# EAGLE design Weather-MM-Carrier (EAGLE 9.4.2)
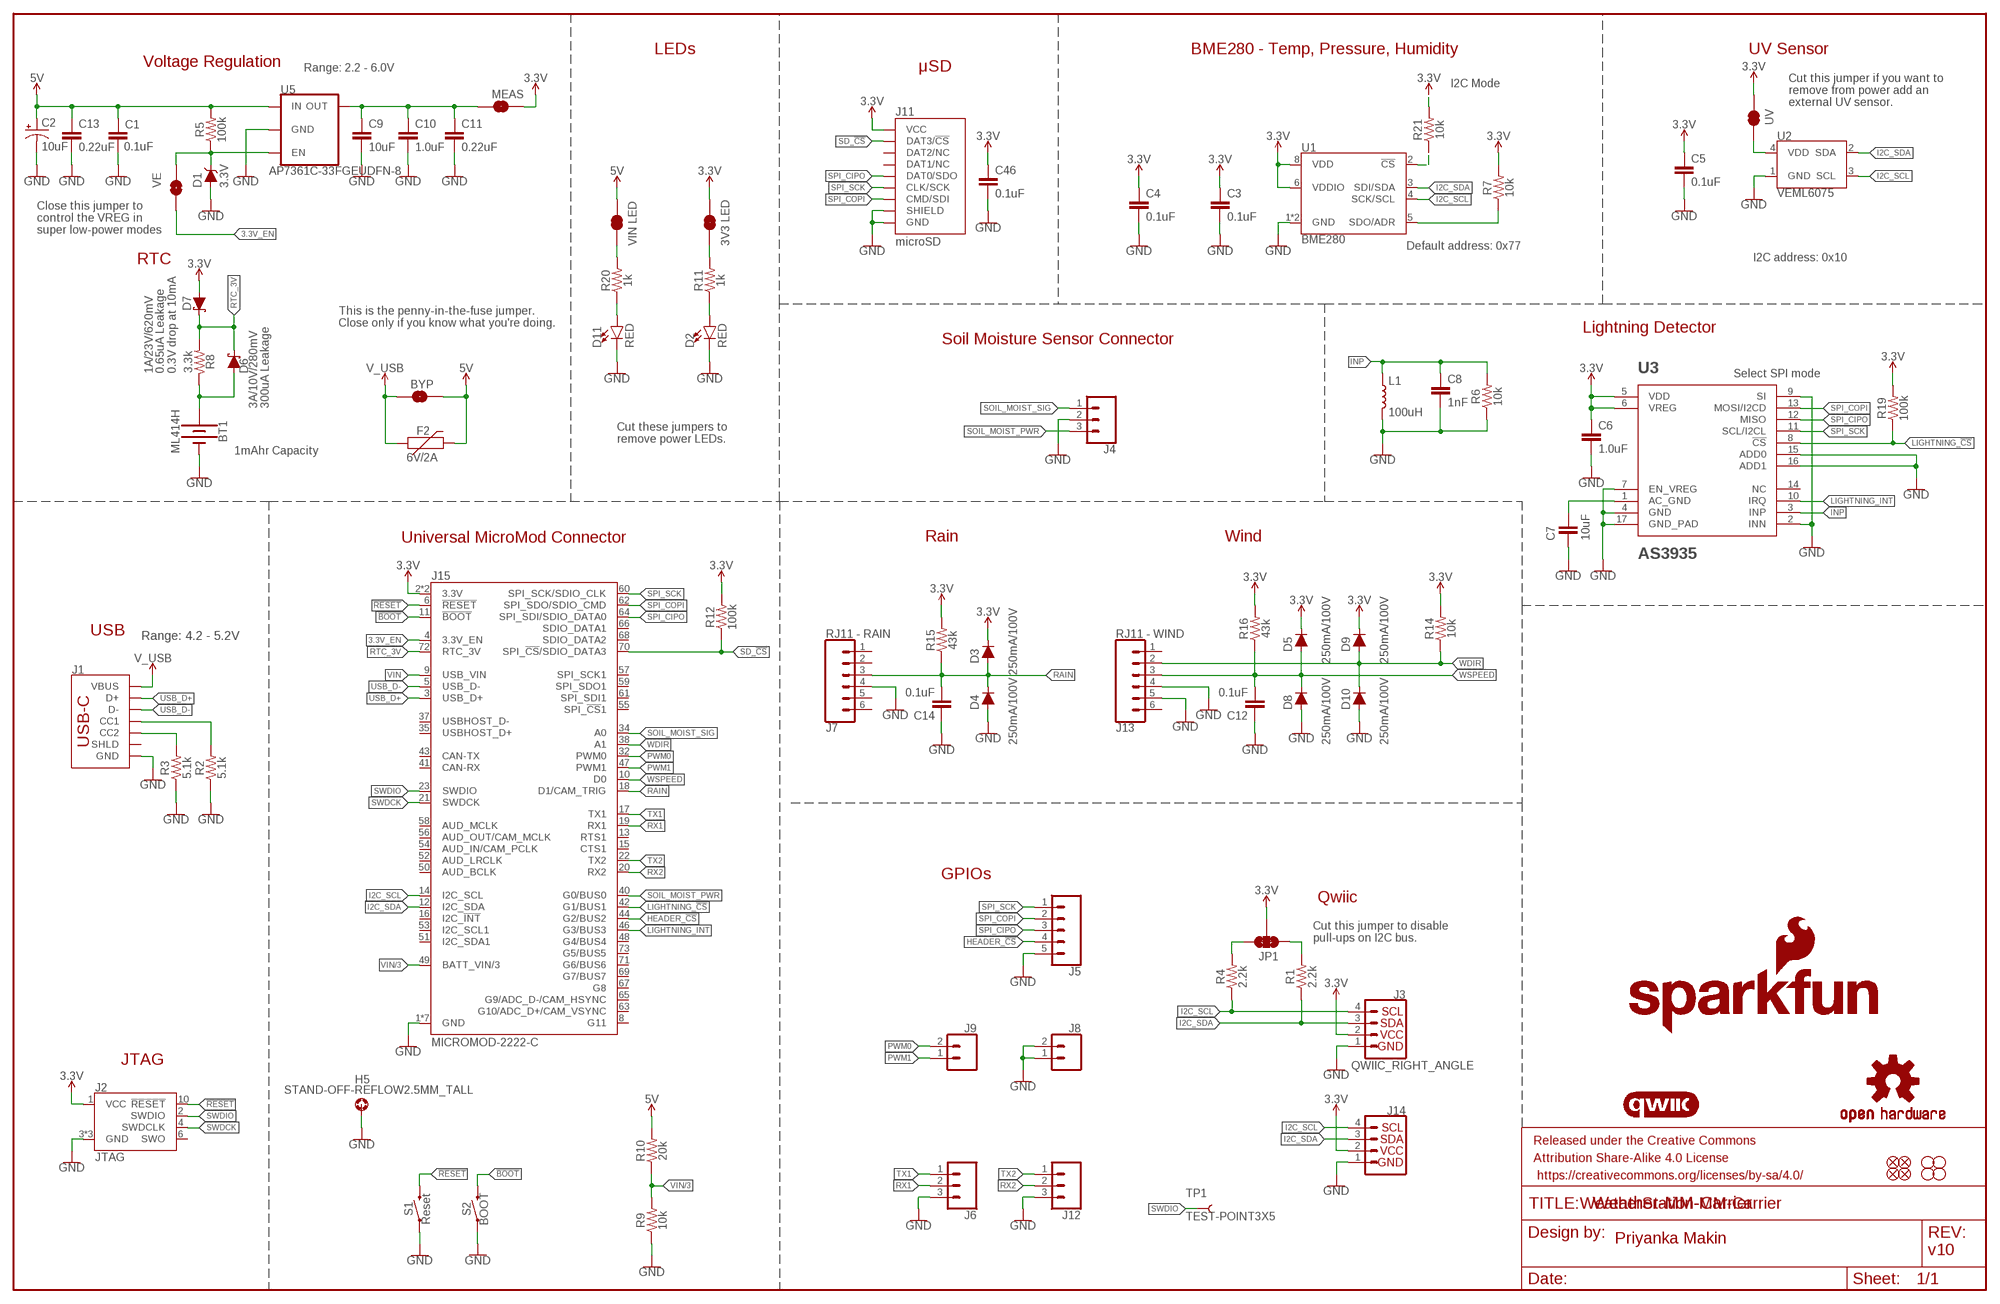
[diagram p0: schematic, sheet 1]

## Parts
BT1  ML414H  ML414H_IV01E_BATTERY  [ML414H_IV01E]
BYP  JUMPER-SMT_2_NO_SILK  [SMT-JUMPER_2_NO_SILK]
C1  0.1uF  0.1UF-0603-25V-(+80/-20%)  [0603]
C2  10uF  10UF-POLAR-EIA3216-16V-10%(TANT)  [EIA3216]
C3  0.1uF  0.1UF-0603-100V-10%  [0603]
C4  0.1uF  0.1UF-0603-100V-10%  [0603]
C5  0.1uF  0.1UF-0603-25V-(+80/-20%)  [0603]
C6  1.0uF  1.0UF-0603-16V-10%  [0603]
C7  10uF  10UF-0603-6.3V-20%  [0603]
C8  1nF  1.0NF/1000PF-0603-50V-10%  [0603]
C9  10uF  10UF-0603-6.3V-20%  [0603]
C10  1.0uF  1.0UF-0603-16V-10%  [0603]
C11  0.22uF  0.22UF-0603-25V-10%  [0603]
C12  0.1uF  0.1UF-0603-25V-(+80/-20%)  [0603]
C13  0.22uF  0.22UF-0603-25V-10%  [0603]
C14  0.1uF  0.1UF-0603-25V-(+80/-20%)  [0603]
C46  0.1uF  0.1UF-0603-25V-(+80/-20%)  [0603]
D1  3.3V  DIODE-ZENER-MM3Z3V3T1G  [SOD-323]
D2  RED  LED-RED0603  [LED-0603]
D3  250mA/100V  DIODE-BAS16J  [SOD-323]
D4  250mA/100V  DIODE-BAS16J  [SOD-323]
D5  250mA/100V  DIODE-BAS16J  [SOD-323]
D6  3A/10V/280mV  DIODE-SCHOTTKY-BAT60A  [SOD-323]
D7  1A/23V/620mV  DIODE-SCHOTTKY-BAT20J  [SOD-323]
D8  250mA/100V  DIODE-BAS16J  [SOD-323]
D9  250mA/100V  DIODE-BAS16J  [SOD-323]
D10  250mA/100V  DIODE-BAS16J  [SOD-323]
D11  RED  LED-RED0603  [LED-0603]
F2  6V/2A  PPTC_6V2A  [1210]
FD1  FIDUCIALUFIDUCIAL  [FIDUCIAL-MICRO]
FD2  FIDUCIALUFIDUCIAL  [FIDUCIAL-MICRO]
FD3  FIDUCIALUFIDUCIAL  [FIDUCIAL-MICRO]
FD4  FIDUCIALUFIDUCIAL  [FIDUCIAL-MICRO]
FRAME1  FRAME-LEDGER  [CREATIVE_COMMONS]
H1  STAND-OFF  [STAND-OFF]
H2  STAND-OFF  [STAND-OFF]
H3  STAND-OFF  [STAND-OFF]
H4  STAND-OFF  [STAND-OFF]
H5  STAND-OFF-REFLOW2.5MM_TALL  [STAND-OFF-REFLOW-M2.5]
J1  USB_C_2-LAYER_PADS  [USB-C-16P-2LAYER-PADS]
J2  JTAG  CORTEX_JTAG_DEBUG_MINIMUM_PTH  [2X5-PTH-1.27MM]
J3  QWIIC_RIGHT_ANGLE  QWIIC_CONNECTORJS-1MM  [JST04_1MM_RA]
J4  CONN_03LATCH  [LATCHTERMINAL-5MM-3]
J5  CONN_05NO_SILK  [1X05_NO_SILK]
J6  CONN_031X03_NO_SILK  [1X03_NO_SILK]
J7  RJ11 - RAIN  RJ11-6  [RJ11-6]
J8  CONN_021X02_NO_SILK  [1X02_NO_SILK]
J9  CONN_021X02_NO_SILK  [1X02_NO_SILK]
J11  microSD  MICRO-SD-SDIOPUSH-PUSH  [MICRO-SD-SOCKET]
J12  CONN_031X03_NO_SILK  [1X03_NO_SILK]
J13  RJ11 - WIND  RJ11-6  [RJ11-6]
J14  I2C_STANDARD_NO_SILK  [1X04_NO_SILK]
J15  MICROMOD-2222-C  [M.2-CONNECTOR-E]
JP1  JUMPER-SMT_3_2-NC_TRACE_SILK  [SMT-JUMPER_3_2-NC_TRACE_SILK]
JP2  VIN LED  JUMPER-SMT_2_NC_TRACE_SILK  [SMT-JUMPER_2_NC_TRACE_SILK]
JP3  UV  JUMPER-SMT_2_NC_TRACE_SILK  [SMT-JUMPER_2_NC_TRACE_SILK]
JP4  3V3 LED  JUMPER-SMT_2_NC_TRACE_SILK  [SMT-JUMPER_2_NC_TRACE_SILK]
JP6  VE  JUMPER-SMT_2_NO_SILK  [SMT-JUMPER_2_NO_SILK]
L1  100uH  MA5532-AE  [MA5532-AE]
LOGO1  SFE_LOGO_NAME_FLAME.2_INCH  [SFE_LOGO_NAME_FLAME_.2]
LOGO2  QWIIC_LOGO_CONNECTOR  [QWIIC_5.5MM]
LOGO3  OSHW-LOGOM  [OSHW-LOGO-M]
MEAS  JUMPER-COMBO_2_NC_TRACE  [COMBO-JUMPER_2_NC_TRACE]
R1  2.2k  2.2KOHM-0603-1/10W-1%  [0603]
R2  5.1k  5.1KOHM5.1KOHM-0603-1/10W-1%  [0603]
R3  5.1k  5.1KOHM5.1KOHM-0603-1/10W-1%  [0603]
R4  2.2k  2.2KOHM-0603-1/10W-1%  [0603]
R5  100k  100KOHM-0603-1/10W-1%  [0603]
R6  10k  10KOHM-0603-1/10W-1%  [0603]
R7  10k  10KOHM-0603-1/10W-1%  [0603]
R8  3.3k  3.3KOHM-0603-1/10W-1%  [0603]
R9  10k  10KOHM-0603-1/10W-1%  [0603]
R10  20k  20KOHM-0603-1/10W-1%  [0603]
R11  1k  1KOHM-0603-1/10W-1%  [0603]
R12  100k  100KOHM-0603-1/10W-1%  [0603]
R14  10k  10KOHM-0603-1/10W-1%  [0603]
R15  43k  43KOHM-0603-1/10W-1%  [0603]
R16  43k  43KOHM-0603-1/10W-1%  [0603]
R19  100k  100KOHM-0603-1/10W-1%  [0603]
R20  1k  1KOHM-0603-1/10W-1%  [0603]
R21  10k  10KOHM-0603-1/10W-1%  [0603]
S1  Reset  MOMENTARY-SWITCH-SPST-SMD-5.2-TALL-REDUNDANT  [TACTILE_SWITCH_SMD_5.2MM]
S2  BOOT  MOMENTARY-SWITCH-SPST-SMD-5.2-TALL-REDUNDANT  [TACTILE_SWITCH_SMD_5.2MM]
TP1  TEST-POINT3X5  [PAD.03X.05]
U1  BME280  [LGA-8-2.5X2.5]
U2  VEML6075  [VEML6075_A3OP]
U3  AS3935  AS3935QFN  [16LD_MLPQ]
U5  AP7361C-33FGEUDFN-8  [UDFN-8]

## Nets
3.3V: C3.1 C4.1 C5.1 C6.1 C46.1 D3.C D5.C D7.A D9.C J2.1(VCC) J3.2 J11.VCC J14.2 J15.2(3.3V) J15.74(3.3V) JP1.2 JP3.2 JP4.2 MEAS.2 MEAS.4 R7.2 R12.2 R14.2 R15.2 R16.2 R19.2 R21.2 U1.6(VDDIO) U1.8(VDD) U3.5(VDD) U3.6(VREG)
3.3V_EN: J15.4(3.3V_EN) JP6.1
!BOOT!: J15.11(!BOOT!) S2.3 S2.4
!RESET!: J2.10(!RESET) J15.6(!RESET!) S1.3 S1.4
GND: BT1.- C1.2 C2.- C3.2 C4.2 C5.2 C6.2 C7.2 C8.2 C9.2 C10.2 C11.2 C12.1 C13.2 C14.1 C46.2 D1.A D2.C D4.A D8.A D10.A D11.C H5.1 J1.GND J1.GND2(GND) J2.3(GND) J2.5(GND) J2.9(GND) J3.1 J4.2 J5.5 J6.3 J7.4 J8.1 J8.2 J11.CD1(SHIELD) J11.GND J11.GND1(GND) J11.GND3(GND) J12.3 J13.4 J13.5 J14.1 J15.1(GND) J15.7(GND) J15.33(GND) J15.36(GND) J15.39(GND) J15.45(GND) J15.75(GND) L1.2 R2.1 R3.1 R6.1 R9.1 S1.1 S1.2 S2.1 S2.2 U1.1(GND) U1.7(GND) U2.1(GND) U3.2(INN) U3.4(GND) U3.7(EN_VREG) U3.9(SI) U3.15(ADD0) U3.16(ADD1) U3.17(GND_PAD) U5.4(GND) U5.EP(GND)
HEADER_!CS!: J5.4 J15.44(G2/BUS2)
I2C_SCL: J3.4 J14.4 J15.14(I2C_SCL) R4.1 U1.4(SCK/SCL) U2.3(SCL)
I2C_SDA: J3.3 J14.3 J15.12(I2C_SDA) R1.1 U1.3(SDI/SDA) U2.2(SDA)
INP: C8.1 L1.1 R6.2 U3.3(INP)
LIGHTNING_!CS!: J15.42(G1/BUS1) R19.1 U3.8(!CS)
LIGHTNING_INT: J15.46(G3/BUS3) U3.10(IRQ)
N$1: C9.1 C10.1 C11.1 MEAS.1 MEAS.3 U5.1(OUT)
N$2: JP1.3 R4.2
N$3: JP1.1 R1.2
N$4: JP4.1 R11.2
N$5: JP2.1 R20.2
N$6: D2.A R11.1
N$7: JP3.1 U2.4(VDD)
N$8: R7.1 U1.5(SDO/ADR)
N$10: J1.A5(CC1) R2.2
N$11: J1.B5(CC2) R3.2
N$14: BT1.+ D6.A R8.1
N$15: C7.1 U3.1(AC_GND)
N$16: D11.A R20.1
N$19: R21.1 U1.2(!CS)
PWM0: J9.2 J15.32(PWM0)
PWM1: J9.1 J15.47(PWM1)
RAIN: C14.2 D3.A D4.C J7.3 J15.18(D1/CAM_TRIG) R15.1
RTC_3V: D6.C D7.C J15.72(RTC_3V) R8.2
RX1: J6.2 J15.19(RX1)
RX2: J12.2 J15.20(RX2)
SD_!CS!: J11.CS/DAT3(DAT3/!CS!) J15.70(SPI_!CS!/SDIO_DATA3) R12.1
SOIL_MOIST_PWR: J4.3 J15.40(G0/BUS0)
SOIL_MOIST_SIG: J4.1 J15.34(A0)
SPI_CIPO: J5.3 J11.DO/DAT0(DAT0/SDO) J15.64(SPI_SDI/SDIO_DATA0) U3.12(MISO)
SPI_COPI: J5.2 J11.DI/CMD(CMD/SDI) J15.62(SPI_SDO/SDIO_CMD) U3.13(MOSI/I2CD)
SPI_SCK: J5.1 J11.SCLK(CLK/SCK) J15.60(SPI_SCK/SDIO_CLK) U3.11(SCL/I2CL)
SWDCK: J2.4(SWDCLK) J15.21(SWDCK)
SWDIO: J2.2(SWDIO) J15.23(SWDIO) TP1.P$1
TX1: J6.1 J15.17(TX1)
TX2: J12.1 J15.22(TX2)
USB_D+: J1.A6(D+) J1.B6(D+) J15.3(USB_D+)
USB_D-: J1.A7(D-) J1.B7(D-) J15.5(USB_D-)
V_USB: BYP.1 F2.1 J1.VBUS1(VBUS) J1.VBUS2(VBUS)
VIN: BYP.2 C1.1 C2.+ C13.1 F2.2 J15.9(USB_VIN) JP2.2 R5.2 R10.2 U5.8(IN) ; supply symbol labelled 5V
VIN/3: J15.49(BATT_VIN/3) R9.2 R10.1
VREG_EN: D1.C JP6.2 R5.1 U5.5(EN)
WDIR: D9.A D10.C J13.2 J15.38(A1) R14.1
WSPEED: C12.2 D5.A D8.C J13.3 J15.10(D0) R16.1
Unconnected: J1.SHLD1(SHLD) J1.SHLD2(SHLD) J1.SHLD3(SHLD) J1.SHLD4(SHLD) J2.6(SWO) J7.1 J7.2 J7.5 J7.6 J11.DAT1(DAT1/NC) J11.DAT2(DAT2/NC) J13.1 J13.6 J15.8(G11) J15.13(RTS1) J15.15(CTS1) J15.16(I2C_!INT!) J15.35(USBHOST_D+) J15.37(USBHOST_D-) J15.41(CAN-RX) J15.43(CAN-TX) J15.48(G4/BUS4) J15.50(AUD_BCLK) J15.51(I2C_SDA1) J15.52(AUD_LRCLK) J15.53(I2C_SCL1) J15.54(AUD_IN/CAM_PCLK) J15.55(SPI_!CS!1) J15.56(AUD_OUT/CAM_MCLK) J15.57(SPI_SCK1) J15.58(AUD_MCLK) J15.59(SPI_SDO1) J15.61(SPI_SDI1) J15.63(G10/ADC_D+/CAM_VSYNC) J15.65(G9/ADC_D-/CAM_HSYNC) J15.66(SDIO_DATA1) J15.67(G8) J15.68(SDIO_DATA2) J15.69(G7/BUS7) J15.71(G6/BUS6) J15.73(G5/BUS5) U3.14(NC)

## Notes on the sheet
- LEDs | BME280 - Temp, Pressure, Humidity | UV Sensor
- Voltage Regulation
- Range: 2.2 - 6.0V | μSD
- I2C Mode
- Cut this jumper if you want to
  remove from power add an 
  external UV sensor.
- Close this jumper to 
  control the VREG in 
  super low-power modes
- Default address: 0x77
- RTC | I2C address: 0x10
- This is the penny-in-the-fuse jumper.
  Close only if you know what you're doing.
- Lightning Detector
- Soil Moisture Sensor Connector
- 0.65uA Leakage
  0.3V drop at 10mA
- Select SPI mode
- 300uA Leakage
- Cut these jumpers to
  remove power LEDs.
- 1mAhr Capacity
- Universal MicroMod Connector | Rain | Wind
- USB
- Range: 4.2 - 5.2V
- GPIOs
- Qwiic
- Cut this jumper to disable
  pull-ups on I2C bus.
- JTAG
- WeatherStation-MM-Carrier
- Priyanka Makin
- v10

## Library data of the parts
BT1 = SparkFun-Batteries:ML414H_IV01E_BATTERY: SEIKO ML414H-IV01E Reflowable Lithium Battery; PROD_ID: BATT-14267
BYP JP6 = SparkFun-Jumpers:JUMPER-SMT_2_NO: Normally open jumper
C1 C5 C12 C14 C46 = SparkFun-Capacitors:0.1UF: 0.1µF ceramic capacitors; PROD_ID: CAP-00810
C2 = SparkFun-Capacitors:10UF-POLAR: 10.0µF polarized capacitors; PROD_ID: CAP-00811
C3 C4 = SparkFun-Capacitors:0.1UF: 0.1µF ceramic capacitors; PROD_ID: CAP-08390
C6 C10 = SparkFun-Capacitors:1.0UF: 1µF ceramic capacitors; PROD_ID: CAP-00868
C7 C9 = SparkFun-Capacitors:10UF: 10.0µF ceramic capacitors; PROD_ID: CAP-11015
C8 = SparkFun-Capacitors:1.0NF/1000PF: 1nF/1,000pF ceramic capacitors; PROD_ID: CAP-07886
C11 C13 = SparkFun-Capacitors:0.22UF: 0.22µF ceramic capacitors; PROD_ID: CAP-07822
D1 = SparkFun-DiscreteSemi:DIODE-ZENER: Zener Diode; PROD_ID: DIO-11284
D2 D11 = SparkFun-LED:LED-RED: Red SMD LED; PROD_ID: DIO-00819
D3-D5 D8-D10 = SparkFun-DiscreteSemi:DIODE: Diode; PROD_ID: DIO-09646
D6 = SparkFun-DiscreteSemi:DIODE-SCHOTTKY: Schottky diode; PROD_ID: DIO-14072
D7 = SparkFun-DiscreteSemi:DIODE-SCHOTTKY: Schottky diode; PROD_ID: DIO-11623
F2 = SparkFun-Fuses:PPTC: Resettable Fuse PPTC; PROD_ID: RES-14313
FD1-FD4 = SparkFun-Aesthetics:FIDUCIAL: Fiducial Alignment Points
FRAME1 = SparkFun-Aesthetics:FRAME-LEDGER: Schematic Frame - Ledger
H1-H4 = SparkFun-Hardware:STAND-OFF: Stand Off
H5 = SparkFun-Hardware:STAND-OFF-REFLOW: Stand Off Reflow Compatible; PROD_ID: HW-14899
J1 = SparkFun-Connectors:USB_C: USB Type C 16Pin Connector Super Speed pins not available on the 16-pin purely SMD connector so this part is best for USB 2.0 implementations. D1 and D2 are tied together enabling D+/- no matter which way the cable is plugged into the connector. The two channel configuration pins (CC1/2) are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; PROD_ID: CONN-14122
J2 = SparkFun-Connectors:CORTEX_JTAG_DEBUG_MINIMUM: Cortex Debug Connector - 10 pin Supports JTAG debug, Serial Wire debug, and Serial Wire Viewer. PTH and SMD connector options available. General Connector Information Products: PTH Connector -via Digi-Key SparkFun PSoc SparkFun T
J3 = SparkFun-Connectors:QWIIC_CONNECTOR: SparkFun I2C Standard Qwiic Connector An SMD 1mm pitch JST connector makes it easy and quick (get it? Qwiic?) to connect I2C devices to each other. The Qwiic system enables fast and solderless connection between popular platforms and various sensors and actuators. We carry 200mm, 100mm, 50mm, and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; PROD_ID: CONN-13694
J4 = SparkFun-Connectors:CONN_03: Multi connection point. Often used as Generic Header-pin footprint for 0.1 inch spaced/style header connections On any of the 0.1 inch spaced packages, you can populate with these: Break Away Headers - Straight (PRT-00116) Break Away Male Headers - Right Angle (PRT-00553) Female Headers (PRT-00115)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; PROD_ID: CONN-14721
J5 = SparkFun-Connectors:CONN_05: Multi connection point. Often used as Generic Header-pin footprint for 0.1 inch spaced/style header connections On any of the 0.1 inch spaced packages, you can populate with these: Break Away Headers - Straight (PRT-00116) Break Away Male Headers - Right Angle (PRT-00553) Female Headers (PRT-00115)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
J6 J12 = SparkFun-Connectors:CONN_03: Multi connection point. Often used as Generic Header-pin footprint for 0.1 inch spaced/style header connections On any of the 0.1 inch spaced packages, you can populate with these: Break Away Headers - Straight (PRT-00116) Break Away Male Headers - Right Angle (PRT-00553) Female Headers (PRT-00115)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
J7 J13 = SparkFun-Connectors:RJ11-6: RJ11 Jack - 6 pin Commonly found on CAT3 devices and some Microchip programmers. Here is the connector we sell at SparkFun: RJ11 6-Pin Connector (PRT-00132) Datasheet It is used on this SparkFun product: SparkFun Weather Shield (DEV-12081) Weather Meters (SEN-08942); PROD_ID: CONN-08590; SF_ID: PRT-00132; VALUE: RJ11
J8 J9 = SparkFun-Connectors:CONN_02: Multi connection point. Often used as Generic Header-pin footprint for 0.1 inch spaced/style header connections
J11 = SparkFun-Connectors:MICRO-SD-SDIO: microSD Socket for Transflash Push-push type µSD socket. tDoc lines correctly indicate media card edge positions when inserting (unlocked, locked, depressed). NOTE: CD1 and CD2 are connected internally, and the default detect state of the socket is detect pin to ground. SparkFun Products: WAV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; PROD_ID: CONN-07820
J14 = SparkFun-Connectors:I2C_STANDARD: SparkFun I2C Standard Pinout Header SparkFun has standardized on a pinout for all I2C based sensor breakouts. This pinout allows I2C boards to be plugged directly into the headers on Arduino Uno compatible boards, and to be daisy chained easily. Example SparkFun Products: SparkFun Atmospheric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
J15 = SparkFun-MicroMod:MICROMOD: MicroMod Connector Description: A card edge connector and mating PCB connector to allow various MicroMod Processor Boards to be coupled with various carrier boards of different capabilities. Based on the M.2 standard.; PROD_ID: CONN-14877
JP1 = SparkFun-Jumpers:JUMPER-SMT_3_2-NC_TRACE: Normally closed trace jumper (2 of 2 connections) This jumper has a trace between all three pads so they are normally closed (NC). Use a razor knife to open the connection(s). For best results follow the IPC guidelines for cutting traces: Cutout at least 0.063 mm (0.005 in). Remove all loose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
JP2-JP4 = SparkFun-Jumpers:JUMPER-SMT_2_NC_TRACE: Normally closed trace jumper
L1 = SparkFun-Coils:MA5532-AE: RFID Transponder Coil - MA5532-AE; PROD_ID: NDUC-11334
LOGO1 = SparkFun-Aesthetics:SFE_LOGO_NAME_FLAME: SparkFun Font Logo w/ Flame
LOGO2 = SparkFun-Aesthetics:QWIIC_LOGO: Qwiic Logos for placement on schematic and PCB. The 5.5mm silk logo is best for placing next to Qwiic connector.
LOGO3 = SparkFun-Aesthetics:OSHW-LOGO: Open-Source Hardware (OSHW) Logo
MEAS = SparkFun-Jumpers:JUMPER-COMBO_2_NC_TRACE
R1 R4 = SparkFun-Resistors:2.2KOHM: 2.2kΩ resistor; PROD_ID: RES-08272
R2 R3 = SparkFun-Resistors:5.1KOHM; PROD_ID: RES-12083
R5 R12 R19 = SparkFun-Resistors:100KOHM: 100kΩ resistor; PROD_ID: RES-07828
R6 R7 R9 R14 R21 = SparkFun-Resistors:10KOHM: 10kΩ resistor; PROD_ID: RES-00824
R8 = SparkFun-Resistors:3.3KOHM: 3.3kΩ resistor; PROD_ID: RES-07851
R10 = SparkFun-Resistors:20KOHM: 20kΩ resistor; PROD_ID: RES-09383
R11 R20 = SparkFun-Resistors:1KOHM: 1kΩ resistor; PROD_ID: RES-07856
R15 R16 = SparkFun-Resistors:43KOHM: 43kΩ resistor; PROD_ID: RES-07858
S1 S2 = SparkFun-Switches:MOMENTARY-SWITCH-SPST: Momentary Switch (Pushbutton) - SPST; PROD_ID: SWCH-14139
TP1 = SparkFun-Connectors:TEST-POINT: SparkFun Test Points
U1 = SparkFun-Sensors:BME280: Bosch BME280 &ndash; Combined Humidity and Pressure Sensor The BME280 is as combined digital humidity, pressure and temperature sensor based on proven sensing principles. The sensor module is housed in an extremely compact metal-lid LGA package with a footprint of only 2.5×2.5mm² with a height of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; PROD_ID: IC-13090
U2 = SparkFun-Sensors:VEML6075: Vishay VEML6075 UVA and UVB light sensor with I2C interface.; PROD_ID: IC-14149
U3 = SparkFun-Sensors:AS3935: AS3935 Franklin Lightning Sensor The AS3935 is a programmable fully integrated Lightning Sensor IC that detects the presence and approach of potentially hazardous lightning activity in the vicinity and provides an estimation on the distance to the head of the storm. The embedded lightning algorithm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; PROD_ID: IC-11333
U5 = SparkFun-IC-Power:AP7361C-33FGE: AP7361C 3.3V LDO Regulator; PROD_ID: VREG-14094

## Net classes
0 default: width 0 mm, drill 0 mm
1 power: width 0.762 mm

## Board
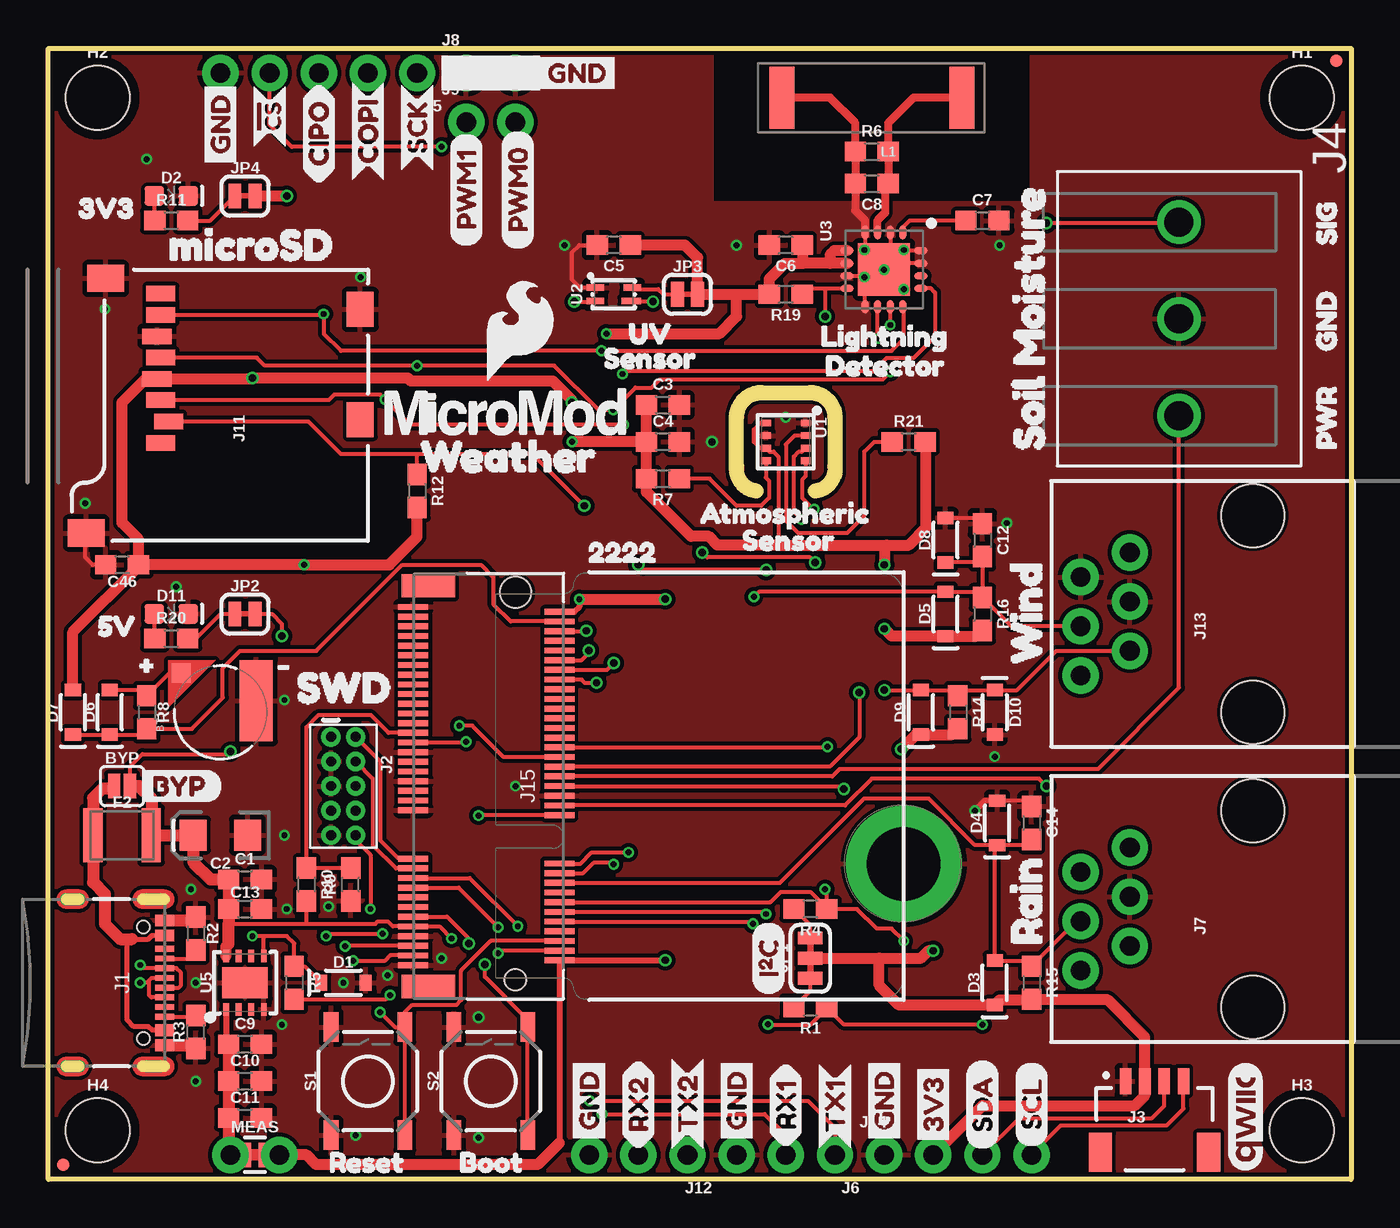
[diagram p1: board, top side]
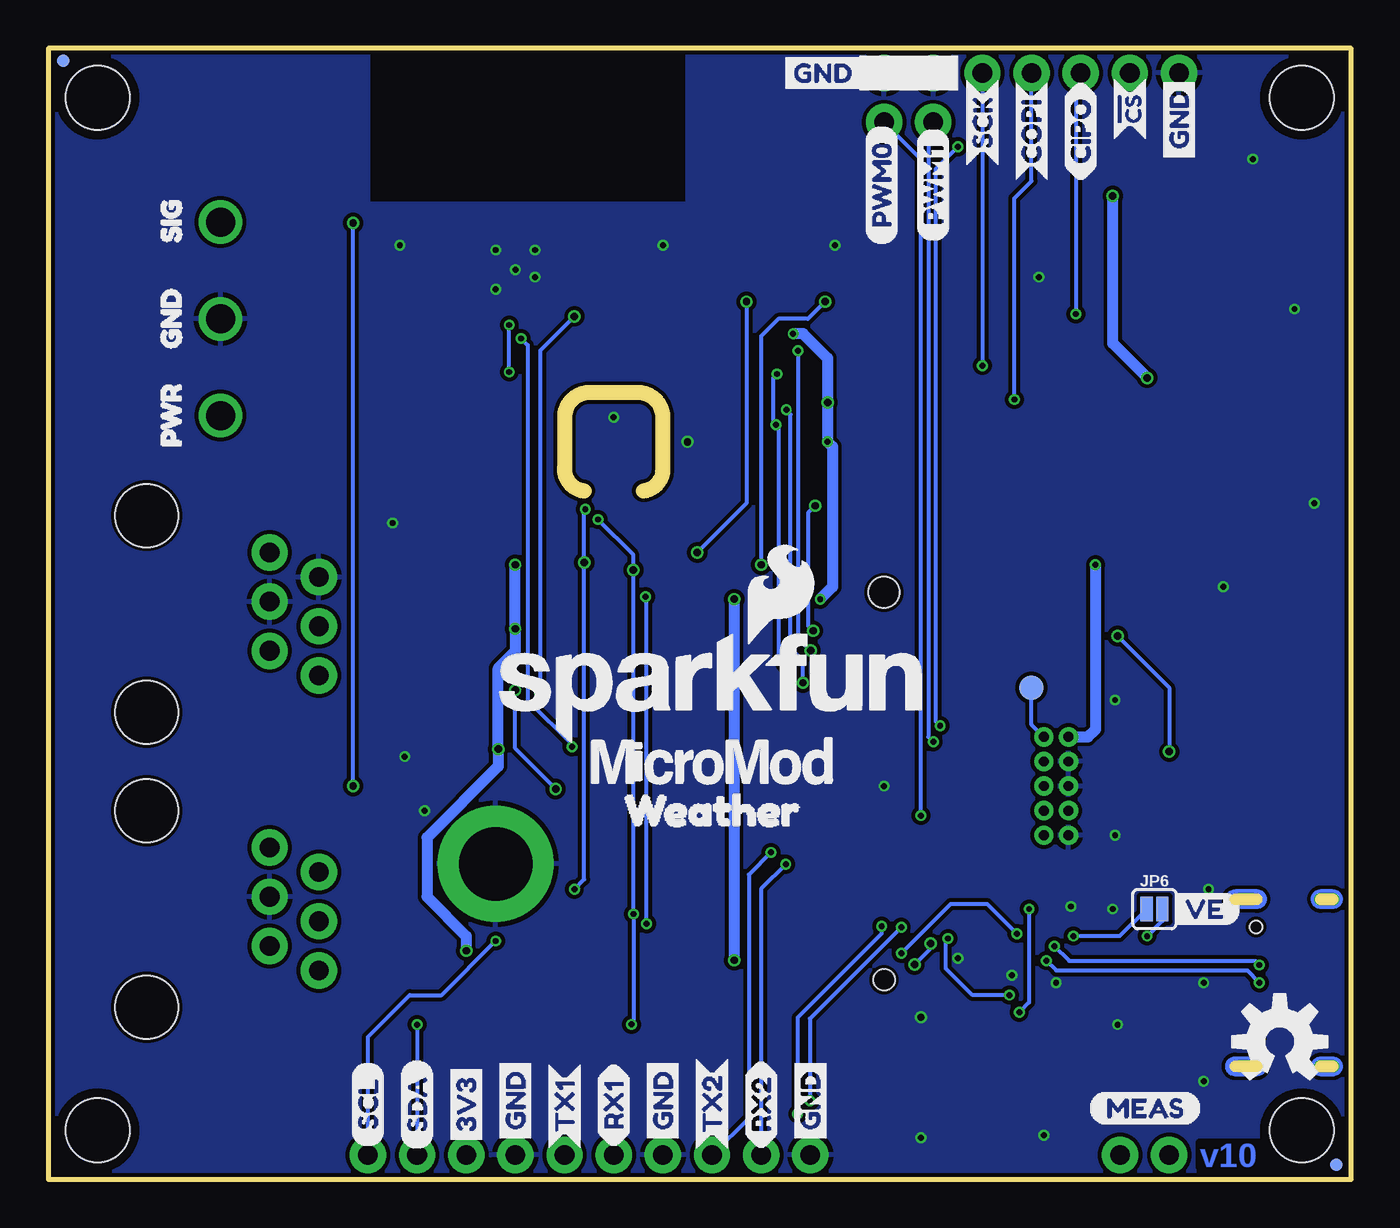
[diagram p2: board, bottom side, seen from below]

Size 67.31 x 58.42 mm. Coordinates in mm from the lower left corner, seen from the top.
Outline: 36.58,35.56 arc-90 35.56,36.83 35.56,39.37 arc-90 36.83,40.64 39.37,40.64 arc-90 40.64,39.37 40.64,36.83 arc-90 39.62,35.56
Outline: 0,0 0,58.42 67.31,58.42 67.31,0 0,0
Copper layers (1*16): Top 0.035mm / dielectric 1.5mm / Bottom 0.035mm
Design rules "SparkFun-2-layer-FAB-LIMIT": minimum track width 4mil, minimum drill 6mil, track to track 4mil, track to pad 4mil, pad to pad 4mil, via to via 4mil, smd to smd 4mil, copper to edge 4mil, drill to drill 4mil, minimum pad ring 5mil, minimum via ring 5mil, stop-mask expansion 4mil, vias tented up to drill 25mil, thermal gap 10mil
tRestrict: 4 lines

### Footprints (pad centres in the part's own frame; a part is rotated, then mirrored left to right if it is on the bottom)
ML414H_IV01E = smd 1 x 1: + 2.022,2.032 | smd 4.2 x 1.7: - 0.6,-1.85
SMT-JUMPER_2_NO_SILK = smd 0.635 x 1.27: 1 -0.406,0; 2 0.406,0
0603 = smd 1.1 x 1: 1 -0.85,0; 2 0.85,0
EIA3216 = smd 1.4 x 1.6: + 1.4,0; - -1.4,0
SOD-323 = smd 0.63 x 0.83: A 1.15,0; C -1.15,0
LED-0603 = smd 1 x 1: A -0.877,0; C 0.877,0
1210 = smd 1 x 2.8: 1 -1.5,0; 2 1.5,0
FIDUCIAL-MICRO = smd 0.635 x 0.635: 1 0,0
STAND-OFF = hole 3.302: 0,0
STAND-OFF-REFLOW-M2.5 = drill 3.8 pad 6: 1 0,0
USB-C-16P-2LAYER-PADS = smd 0.3 x 1: A5 -1.25,-0.34; A6 -0.25,-0.34; A7 0.25,-0.34; A8 1.25,-0.34; B5 1.75,-0.34; B6 0.75,-0.34; B7 -0.75,-0.34; B8 -1.75,-0.34 | smd 0.6 x 1: GND -3.225,-0.34; GND2 3.225,-0.34; VBUS1 -2.45,-0.34; VBUS2 2.45,-0.34 | drill 0.4 pad 0.6 long: SHLD1 -4.318,-0.915; SHLD2 4.318,-0.915; SHLD3 -4.318,-5.095; SHLD4 4.318,-5.095 | hole 0.65: -2.89,-1.445; 2.89,-1.445
2X5-PTH-1.27MM = drill 0.508 pad 1: 1 -2.54,-0.635; 2 -2.54,0.635; 3 -1.27,-0.635; 4 -1.27,0.635; 5 0,-0.635; 6 0,0.635; 7 1.27,-0.635; 8 1.27,0.635; 9 2.54,-0.635; 10 2.54,0.635
JST04_1MM_RA = smd 0.6 x 1.35: 1 -1.5,0; 2 -0.5,0; 3 0.5,0; 4 1.5,0 | smd 1.2 x 2: NC1 2.8,-3.675; NC2 -2.8,-3.675
LATCHTERMINAL-5MM-3 = drill 1.5: 1 -5,0; 2 0,0; 3 5,0
1X05_NO_SILK = drill 1.016 pad 1.88: 1 0,0; 2 2.54,0; 3 5.08,0; 4 7.62,0; 5 10.16,0
1X03_NO_SILK = drill 1.016 pad 1.88: 1 0,0; 2 2.54,0; 3 5.08,0
RJ11-6 = drill 1.016 pad 1.88: 1 -3.175,8.89; 2 -1.905,6.35; 3 -0.635,8.89; 4 0.635,6.35; 5 1.905,8.89; 6 3.175,6.35 | hole 3.251: -5.08,0; 5.08,0
1X02_NO_SILK = drill 1.016 pad 1.88: 1 0,0; 2 2.54,0
MICRO-SD-SOCKET = smd 1.8 x 1.4: CD1 -2.05,0.4; CD2 -7.75,0.4 | smd 0.8 x 1.5: CS/DAT3 -7.84,10.3; DAT1 -1.24,10.7; DAT2 -8.94,10.7; DI/CMD -6.74,10.7; DO/DAT0 -2.34,10.7; GND -3.44,10.9; SCLK -4.54,10.7; VCC -5.64,10.9 | smd 1.4 x 1.9: GND1 -13.6,14.55; GND3 -0.45,13.55
1X04_NO_SILK = drill 1.016 pad 1.88: 1 0,0; 2 2.54,0; 3 5.08,0; 4 7.62,0
M.2-CONNECTOR-E = smd 0.3 x 1.55: 1 9.25,-5.275; 2 9,2.275; 3 8.75,-5.275; 4 8.5,2.275; 5 8.25,-5.275; 6 8,2.275; 7 7.75,-5.275; 8 7.5,2.275; 9 7.25,-5.275; 10 7,2.275; 11 6.75,-5.275; 12 6.5,2.275; 13 6.25,-5.275; 14 6,2.275; 15 5.75,-5.275; 16 5.5,2.275; 17 5.25,-5.275; 18 5,2.275; 19 4.75,-5.275; 20 4.5,2.275; 21 4.25,-5.275; 22 4,2.275; 23 3.75,-5.275; 32 1.5,2.275; 33 1.25,-5.275; 34 1,2.275; 35 0.75,-5.275; 36 0.5,2.275; 37 0.25,-5.275; 38 0,2.275; 39 -0.25,-5.275; 40 -0.5,2.275; 41 -0.75,-5.275; 42 -1,2.275; 43 -1.25,-5.275; 44 -1.5,2.275; 45 -1.75,-5.275; 46 -2,2.275; 47 -2.25,-5.275; 48 -2.5,2.275; 49 -2.75,-5.275; 50 -3,2.275; 51 -3.25,-5.275; 52 -3.5,2.275; 53 -3.75,-5.275; 54 -4,2.275; 55 -4.25,-5.275; 56 -4.5,2.275; 57 -4.75,-5.275; 58 -5,2.275; 59 -5.25,-5.275; 60 -5.5,2.275; 61 -5.75,-5.275; 62 -6,2.275; 63 -6.25,-5.275; 64 -6.5,2.275; 65 -6.75,-5.275; 66 -7,2.275; 67 -7.25,-5.275; 68 -7.5,2.275; 69 -7.75,-5.275; 70 -8,2.275; 71 -8.25,-5.275; 72 -8.5,2.275; 73 -8.75,-5.275; 74 -9,2.275; 75 -9.25,-5.275 | smd 1.2 x 2.75: A1 10.35,-4.5; A2 -10.35,-4.5 | hole 1.1: 10,0 | hole 1.6: -10,0
SMT-JUMPER_3_2-NC_TRACE_SILK = smd 0.66 x 1.27: 1 -1.041,0; 2 0,0; 3 1.041,0
SMT-JUMPER_2_NC_TRACE_SILK = smd 0.66 x 1.27: 1 -0.521,0; 2 0.521,0
MA5532-AE = smd 1.3 x 3.2: 1 -4.65,0; 2 4.65,0
COMBO-JUMPER_2_NC_TRACE = smd 0.635 x 1.27: 1 -0.508,0; 2 0.508,0 | drill 1.016 pad 1.88: 3 -1.27,0; 4 1.27,0
TACTILE_SWITCH_SMD_5.2MM = smd 1.524 x 0.762: 1 -2.794,1.905; 2 2.794,1.905; 3 -2.794,-1.905; 4 2.794,-1.905
PAD.03X.05 = smd 1.27 x 1.27: P$1 0,0
LGA-8-2.5X2.5 = smd 0.35 x 0.5: 1 -0.975,1.025; 2 -0.325,1.025; 3 0.325,1.025; 4 0.975,1.025; 5 0.975,-1.025; 6 0.325,-1.025; 7 -0.325,-1.025; 8 -0.975,-1.025
VEML6075_A3OP = smd 0.9 x 0.35: 1 -0.95,0.35; 2 -0.95,-0.35; 4 0.95,0.35 | smd 1 x 0.35: 3 0.9,-0.35
16LD_MLPQ = smd 0.7 x 0.35: 1 -1.919,0.968; 2 -1.919,0.318; 3 -1.919,-0.332; 4 -1.919,-0.982; 9 1.908,-0.982; 10 1.908,-0.332; 11 1.908,0.318; 12 1.908,0.968 | smd 0.35 x 0.7: 5 -0.982,-1.917; 6 -0.332,-1.917; 7 0.318,-1.917; 8 0.968,-1.917; 13 0.968,1.907; 14 0.318,1.907; 15 -0.332,1.907; 16 -0.982,1.907 | smd 2.7 x 2.7: 17 -0.007,-0.007
UDFN-8 = smd 0.3 x 0.65: 1 -0.975,-1.375; 2 -0.325,-1.375; 3 0.325,-1.375; 4 0.975,-1.375; 5 0.975,1.375; 6 0.325,1.375; 7 -0.325,1.375; 8 -0.975,1.375 | smd 2.35 x 1.6: EP 0,0

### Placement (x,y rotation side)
BT1  8.89,24.13 90 top
BYP  3.81,20.32 0 top
C1  10.16,15.49 0 top
C2  8.89,17.78 180 top
C3  31.75,40.01 0 top
C4  31.75,38.1 0 top
C5  29.21,48.26 180 top
C6  38.1,48.26 180 top
C7  48.26,49.53 0 top
C8  42.55,51.44 180 top
C9  10.16,6.99 0 top
C10  10.16,5.08 0 top
C11  10.16,3.17 0 top
C12  48.26,33.02 270 top
C13  10.16,13.97 0 top
C14  50.8,18.41 270 top
C46  3.81,31.75 180 top
D1  15.24,10.16 0 top
D2  6.35,50.8 0 top
D3  48.9,10.16 90 top
D4  49.02,18.41 90 top
D5  46.35,29.21 90 top
D6  3.17,24.13 90 top
D7  1.27,24.13 90 top
D8  46.35,33.02 90 top
D9  45.09,24.13 90 top
D10  48.9,24.13 270 top
D11  6.35,29.21 0 top
F2  3.81,17.78 0 top
FD1  0.76,0.76 0 top
FD2  66.55,57.78 0 top
FD3  0.76,0.76 0 bottom
FD4  66.55,57.78 0 bottom
FRAME1  not placed on the board
H1  64.77,55.88 0 top
H2  2.54,55.88 0 top
H3  64.77,2.54 0 top
H4  2.54,2.54 0 top
H5  44.2,16.3 0 top
J1  6.35,10.16 270 top
J2  15.24,20.32 270 top
J3  57.15,5.08 0 top
J4  58.42,44.45 270 top
J5  19.05,57.15 180 top
J6  40.64,1.27 180 top
J7  62.23,13.97 90 top
J8  21.59,57.15 0 top
J9  21.59,54.61 0 top
J11  16.51,46.99 90 top
J12  33.02,1.27 180 top
J13  62.23,29.21 90 top
J14  43.18,1.27 0 top
J15  24.13,20.32 270 top
JP1  39.37,11.43 90 top
JP2  10.16,29.21 0 top
JP3  33.02,45.72 0 top
JP4  10.16,50.8 0 top
JP6  10.16,13.97 0 bottom
L1  42.55,55.88 180 top
LOGO1  33.02,25.4 0 bottom
LOGO2  61.85,3.24 90 top
LOGO3  3.68,7.11 0 bottom
MEAS  10.67,1.27 0 top
R1  39.37,8.89 180 top
R2  7.62,12.7 270 top
R3  7.62,7.62 90 top
R4  39.37,13.97 180 top
R5  12.7,10.16 270 top
R6  42.55,53.09 0 top
R7  31.75,36.2 180 top
R8  5.08,24.13 270 top
R9  15.62,15.24 90 top
R10  13.34,15.24 270 top
R11  6.35,49.53 0 top
R12  19.05,35.56 270 top
R14  46.99,24.13 270 top
R15  50.8,10.16 270 top
R16  48.26,29.21 270 top
R19  38.1,45.72 180 top
R20  6.35,27.94 0 top
R21  44.45,38.1 0 top
S1  16.51,5.08 90 top
S2  22.86,5.08 90 top
TP1  16.51,25.4 0 bottom
U1  38.1,38.1 270 top
U2  29.21,45.72 0 top
U3  43.18,46.99 270 top
U5  10.16,10.16 0 top
U$1  [3V31]  0.64,50.16 0 top
U$2  [RESET3]  13.59,0.89 0 top
U$3  [RAIN1]  50.55,10.79 90 top
U$4  [GND0]  66.04,41.91 90 top
U$5  [MEAS]  13.59,3.68 0 bottom
U$6  [GND_P]  8.89,52.07 90 top
U$7  [COPI0]  16.51,51.56 90 top
U$8  [COPI0]  16.51,51.56 90 bottom
U$9  [SCK_O]  19.05,52.07 90 top
U$10  [!CS_O]  11.43,53.09 90 top
U$11  [GND_P]  29.72,57.15 0 bottom
U$12  [PWR2]  66.04,36.83 90 top
U$13  [SIG1]  66.04,47.37 90 top
U$14  [BYP0]  4.45,20.32 0 top
U$15  [PWM10]  21.59,48.39 90 bottom
U$16  [WEATHER4]  17.91,37.34 0 top
U$17  [RX25]  30.48,1.52 90 top
U$18  [5V0]  1.65,28.57 0 top
U$19  [BOOT2]  20.32,0.89 0 top
U$20  [ATMOSPHERIC0]  32.77,34.42 0 top
U$21  [VE0]  9.53,13.97 0 bottom
U$22  [LIGHTNING8]  38.99,43.56 0 top
U$23  [GND_P]  27.94,1.65 90 bottom
U$24  [PWR2]  60.96,36.96 90 bottom
U$25  [RX10]  38.1,1.65 90 bottom
U$27  [CIPO0]  13.97,51.44 90 top
U$28  [TX24]  33.02,1.52 90 bottom
U$29  [RX10]  38.1,1.65 90 top
U$30  [RX25]  30.48,1.52 90 bottom
U$31  [TX13]  40.64,1.52 90 top
U$32  [GND_P]  35.56,1.65 90 top
U$33  [GND_P]  27.94,1.65 90 top
U$34  [SENSOR7]  27.69,42.42 0 top
U$35  [MICROSD0]  4.83,48.26 0 top
U$36  [GND_P]  43.18,1.65 90 top
U$37  [I2C]  37.21,9.53 90 top
U$38  [3V3_P]  45.72,1.52 90 top
U$39  [SDA_IO]  48.26,1.52 90 top
U$40  [SCL_IO]  50.8,1.65 90 top
U$41  [TX13]  40.64,1.52 90 bottom
U$42  [GND_P]  35.56,1.65 90 bottom
U$43  [SWD1]  11.43,25.4 0 top
U$44  [SFE_LOGO_FLAME_.2]  24.38,43.81 0 top
U$45  [GND_P]  43.18,1.65 90 bottom
U$46  [3V3_P]  45.72,1.52 90 bottom
U$47  [SDA_IO]  48.26,1.52 90 bottom
U$48  [SCL_IO]  50.8,1.65 90 bottom
U$49  [SCK_O]  19.05,52.32 90 bottom
U$50  [CIPO0]  13.97,51.56 90 bottom
U$52  [!CS_O]  11.43,53.47 90 bottom
U$53  [GND_P]  8.89,52.32 90 bottom
U$54  [GND_P]  24.89,57.15 0 top
U$55  [22229]  26.96,32.39 0 top
U$56  [TX24]  33.02,1.52 90 top
U$57  [GND0]  60.96,42.04 90 bottom
U$58  [WEATHER4]  38.86,19.05 0 bottom
U$59  [PWM01]  24.26,48.26 90 bottom
U$60  [PWM01]  24.26,48.01 90 top
U$61  [PWM10]  21.59,48.13 90 top
U$62  [UV6]  29.08,43.69 0 top
U$63  [SIG1]  60.96,47.5 90 bottom
U$64  [SENSOR1]  34.92,33.02 0 top
U$65  [SOIL_MOISTURE2]  50.67,36.32 90 top
U$66  [WIND0]  50.55,25.27 90 top
U$67  [MICROMOD_LOGO_.5]  23.62,39.62 0 top
U$68  [MICROMOD_LOGO_.5]  33.02,21.59 0 bottom
U$69  [#0]  3.81,26.67 0 top
U$70  [#1]  10.92,26.67 0 top
U$71  [DETECTOR2]  39.24,42.04 0 top

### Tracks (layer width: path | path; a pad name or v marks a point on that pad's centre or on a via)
3.3V  (via drill 0.3, 0.38)
  Top 0.203: C46.1 4.7,31.71 4.74,31.75 | 46.69,22.98 R14.2 | 47.96,28.06 R16.2 | U1.8 36.79,39.08 36.45,38.73 36.45,38.1 36.77,37.77 U1.6 37.26,37.59 37.47,37.59 37.72,37.34 37.72,32.77 | v27.05,38.1 27.06,38.11 | 30.89,38.11 C4.1 | 45.34,38.06 R21.2 | D9.C 44.82,22.98 | 38.95,47.36 38.99,47.32
  Top 0.305: 26.41,1.89 J15.2 v31.88,11.32 | J15.74 27.16,29.32 27.43,29.59 v27.43,29.97
  Top 0.559: D7.A 1.27,28.28 4.7,31.71 | 4.74,31.75 v13.21,31.75 17.61,31.75 19.05,33.19 R12.2 | U3.6 40.39,47.32 | 40.39,47.32 38.99,47.32 38.05,47.32 37.25,46.52 R19.2 35.56,45.72 | U3.5 40.61,47.97 40.39,47.75 40.39,47.32 | J14.2 48.26,3.81 56.13,3.81 56.65,4.33 J3.2 56.65,7.36 54.74,9.27 50.84,9.27 | 26.41,1.89 25.27,0.76 13.84,0.76 13.34,1.27 11.56,1.27 | JP1.2 42.93,11.43 | 42.93,11.43 45.09,11.43 45.47,11.81 v45.72,11.81 | D9.C 46.69,22.98 | 47.96,28.06 D5.C 43.58,28.06 v43.19,28.45 | C3.1 C4.1 R7.2 30.9,35.52 33.21,33.21 34.12,33.21 34.57,32.77 37.72,32.77 43.31,32.77 | 30.89,38.11 27.06,38.11 | 45.34,38.06 45.34,33.66 44.45,32.77 43.31,32.77 | 44.82,22.98 v44.07,22.23 | C6.1 38.95,47.36 | v27.05,40.13 27.05,40.26 26.06,41.25 18.72,41.25 18.57,41.4 v10.54,41.4 10.49,41.35 J11.VCC 5.03,41.35 3.81,40.13 3.81,33.91 4.66,33.06 C46.1 | 35.56,45.72 JP3.2 33.54,47.61 32.89,48.26 C5.1 | v28.83,43.69 34.67,43.69 35.56,44.58 35.56,45.72 | 50.84,9.27 R15.2 | 42.93,11.43 42.93,10.03 43.95,9.01 D3.C 49.16,9.27 50.84,9.27 | 43.31,32.77 43.19,32.65 v43.19,31.75 | v27.43,29.97 v31.88,29.97 | JP4.2 v12.32,50.8
  Top 0.61: MEAS.2 11.56,1.27 MEAS.4
  Bottom 0.559: J2.1 13.59,22.86 13.21,23.24 v13.21,31.75 | v27.43,29.97 26.8,30.61 26.8,37.85 v27.05,38.1 v27.05,40.13 27.05,42.42 28.32,43.69 v28.83,43.69 | v45.72,11.81 45.72,12.57 47.75,14.61 47.75,17.65 44.07,21.34 v44.07,22.23 44.07,26.42 43.18,27.3 43.18,28.43 v43.19,28.45 v43.19,31.75 | v31.88,29.97 v31.88,11.32 | v12.32,50.8 12.32,43.18 v10.54,41.4
3.3V_EN  (via drill 0.3)
  Top 0.203: v23.24,11.68 23.38,11.82 J15.4 | v17.27,12.7 14.48,12.7 v14.35,12.57
  Bottom 0.203: v17.27,12.7 18.8,14.22 20.7,14.22 v23.24,11.68 | JP6.1 11.96,12.57 v14.35,12.57
!BOOT!  (via drill 0.38)
  Top 0.203: v22.56,11.1 22.56,10.46 24.77,8.26 S2.4 S2.3 | v21.73,12.19 21.73,12.43 20.59,13.57 J15.11
  Bottom 0.203: v21.73,12.19 21.73,11.93 v22.56,11.1
!RESET!  (via drill 0.3)
  Top 0.203: J2.10 15.88,17.53 16.64,16.76 v16.64,13.97 | v17.14,8.64 17.91,7.87 S1.4 | S1.4 18.41,8.64 18.8,9.02 21.08,9.02 21.34,9.27 21.34,10.79 22.86,12.32 J15.6 | S1.4 S1.3
  Bottom 0.203: v16.64,13.97 16.64,9.14 v17.14,8.64
GND  (via drill 0.3, 0.38)
  Top 0.203: C46.2 2.29,31.75 1.91,32.13 1.91,33.34 J11.GND1 | U3.4 42.2,48.17 | U3.2 43.5,48.2 | U3.16 44.36,47.97 | U3.15 44.37,47.32 | C14.1 50.5,19.57 D4.A | D8.A 47.96,34.17 C12.1 | U3.9 42.2,46.58 v42.16,46.61 42.1,46.67 U3.7 | U2.1 27.46,46.07 27.05,46.48 27.05,47.88 27.43,48.26 C5.2
  Top 0.305: D4.A 48.39,19.57 v47.88,19.05
  Top 0.406: L1.2 40.39,55.88 41.7,54.57 R6.1 C8.2 41.7,50.05 42.2,49.54 U3.4
  Top 0.61: J1.GND2 7.46,6.93 R3.1 | J1.GND 7.46,13.38 R2.1
  other vias: 38.1,39.37 42.16,48.01 43.18,46.99 44.2,48.01 44.2,45.97 12.32,13.97 15.24,10.16 24.13,20.32 20.32,11.43 17.53,10.54 7.62,5.08 7.37,14.99 14.48,14.1 22.23,8.38 34.29,38.1 12.19,17.78 12.06,8 15.88,2.29 22.23,2.16 7.62,10.16 6.6,30.61 12.19,24.77 1.91,34.92 2.92,44.96 5.08,52.7 16.13,46.61 26.67,48.26 35.56,48.26 49.15,48.26 49.53,33.91 48.9,21.84
  pour Top (isolate 0.203): 0,58.42 0,0 67.31,0 67.31,58.42 50.8,58.42 50.8,50.42 34.29,50.42 34.29,58.42
  pour Bottom (isolate 0.203): 0,58.42 0,0 67.31,0 67.31,58.42 50.8,58.42 50.8,50.42 34.29,50.42 34.29,58.42
HEADER_!CS!  (via drill 0.3)
  Top 0.203: J15.44 23.52,21.82 21.9,23.44 v21.23,23.44 | v20.32,53.34 12.57,53.34 11.43,54.48 J5.4
  Bottom 0.203: v21.23,23.44 21.46,23.66 21.46,52.2 v20.32,53.34
I2C_SCL  (via drill 0.3, 0.38)
  Top 0.203: J14.4 52.32,2.79 57.78,2.79 58.65,3.66 J3.4 | v44.2,12.32 43.56,12.95 42.8,12.95 41.78,13.97 R4.1 | R4.1 40.22,14.01 39.37,14.86 37.85,14.86 37.31,14.32 J15.14 | U1.4 39.12,36.33 38.96,36.17 38.96,35.18 39.53,34.62 v39.57,34.62 | R4.1 40.22,14.9 v40.13,14.99 | v31.24,45.34 31.21,45.37 U2.3 | v39.62,31.86 39.36,32.13 34.04,32.13 v33.78,32.38
  Bottom 0.203: J14.4 50.8,7.37 48.64,9.53 46.99,9.53 v44.2,12.32 | v40.13,14.99 39.62,15.49 v39.62,31.86 39.62,34.56 v39.57,34.62 | v31.24,45.34 31.24,34.92 v33.78,32.38
I2C_SDA  (via drill 0.3, 0.38)
  Top 0.203: J14.3 50.16,3.17 57.02,3.17 57.65,3.8 J3.3 | v48.26,8 41.11,8 R1.1 40.22,8.85 39.37,8 v37.18,8 v37.18,8.01 | v37.08,13.71 36.97,13.82 J15.12 | U1.3 38.93,37.58 38.76,37.58 38.52,37.34 38.52,34.48 v38.91,34.09 | v30.48,31.75 30.75,31.48 v37.08,31.48 | U2.2 28.23,45.34 v27.18,45.34
  Bottom 0.203: v48.26,8 J14.3 | v37.18,8.01 37.08,8.1 v37.08,13.71 v37.08,31.48 37.08,32.26 v38.91,34.09 | v27.18,45.34 28.07,44.45 29.59,44.45 30.48,43.56 v30.48,31.75
INP
  Top 0.203: 43.23,51.27 C8.1
  Top 0.406: 43.23,51.27 43.23,49.92 42.85,49.54 U3.3 | C8.1 R6.2 43.4,54.57 44.7,55.88 L1.1
LIGHTNING_!CS!  (via drill 0.38)
  Top 0.203: R19.1 39.25,46.02 40.13,46.02 | 40.13,46.02 U3.8 | 40.13,46.02 v40.13,44.58 | v41.9,25.16 41.9,22.85 40.37,21.32 J15.42
  Bottom 0.203: v40.13,44.58 41.9,42.81 v41.9,25.16
LIGHTNING_INT  (via drill 0.3)
  Top 0.203: J15.46 40.23,22.32 v40.26,22.35 | v42.89,43.43 42.85,43.47 U3.10
  Bottom 0.203: v40.26,22.35 40.26,22.48 42.55,24.77 42.55,43.09 v42.89,43.43
N$1
  Top 0.305: U5.1 9.19,7.11
  Top 0.61: 9.19,7.11 C9.1 C10.1 C11.1 9.31,1.36 MEAS.3 MEAS.1
N$2
  Top 0.203: JP1.3 39.37,13.12 R4.2
N$3
  Top 0.203: R1.2 39.37,9.74 JP1.1
N$4
  Top 0.203: JP4.1 8.37,49.53 R11.2
N$5
  Top 0.203: R20.2 7.62,27.94 8.89,29.21 JP2.1
N$6
  Top 0.203: D2.A 5.47,49.56 R11.1
N$7
  Top 0.203: JP3.1 31.78,45.72 31.51,45.99 30.24,45.99 U2.4
N$8
  Top 0.203: U1.5 37.08,36.25 37.24,36.09 37.24,35.2 36.83,34.8 35.56,34.8 34.16,36.2 R7.1
N$10
  Top 0.203: J1.A5 7.18,11.41 R2.2
N$11
  Top 0.203: J1.B5 7.56,8.41 R3.2
N$14
  Top 0.203: BT1.+ 6.25,26.15 R8.1 4.78,25.28 D6.A
N$15
  Top 0.203: C7.1 44.49,49.53 44.15,49.19 U3.1
N$16
  Top 0.203: D11.A 5.47,27.97 R20.1
N$19
  Top 0.203: U1.2 38.55,38.42 38.1,37.97 38.1,34.04 38.73,33.4 41.27,33.4 42.16,34.29 42.16,37.59 42.67,38.1 R21.1
PWM0  (via drill 0.3)
  Top 0.203: J15.32 22.25,18.82 v22.23,18.8
  Bottom 0.203: v22.23,18.8 22.23,52.7 J9.2
PWM1  (via drill 0.3)
  Top 0.203: J15.47 21.55,22.57 v21.59,22.61
  Bottom 0.203: v21.59,22.61 21.84,22.86 21.84,54.36 J9.1
RAIN
  Top 0.203: J7.3 53.12,13.34 R15.1 50.5,11.31 D3.A 48.9,17.14 D4.C | C14.2 50.5,17.27 D4.C | J15.18 37.8,15.32 42.16,19.68 45.46,19.68 47.88,17.27 D4.C
RTC_3V
  Top 0.203: D7.C D6.C 4.78,22.98 R8.2 7.41,23.28 9.02,24.89 9.02,26.42 9.91,27.3 13.84,27.3 18.29,31.75 22.35,31.75 22.99,31.11 22.99,29.72 23.89,28.82 J15.72
RX1  (via drill 0.3)
  Top 0.203: v24.26,13.08 21.77,15.57 J15.19 | v28.6,3.38 37.01,3.38 38.1,2.29 J6.2
  Bottom 0.203: v24.26,13.08 24.26,12.7 28.6,8.36 v28.6,3.38
RX2  (via drill 0.3)
  Top 0.203: v29.21,16.28 29.11,16.38 28.19,16.38 27.63,15.82 J15.20
  Bottom 0.203: v29.21,16.28 30.48,15.01 J12.2
SD_!CS!  (via drill 0.38)
  Top 0.203: J11.CS/DAT3 13.43,39.15 15.11,37.47 19.05,37.47 | v27.69,34.8 25.02,37.47 19.05,37.47 | J15.70 27.78,28.32 v27.8,28.34 | R12.1 19.05,37.47
  Bottom 0.203: v27.8,28.34 28.05,28.59 28.05,34.43 v27.69,34.8 | v27.69,34.8
SOIL_MOIST_PWR
  Top 0.203: J15.40 40.5,20.82 40.88,21.2 54.22,21.2 58.42,25.4 J4.3
SOIL_MOIST_SIG  (via drill 0.38)
  Top 0.203: v51.56,20.32 51.18,20.7 42.55,20.7 41.16,19.32 J15.34 | v51.56,49.4 58.37,49.4 J4.1
  Bottom 0.203: v51.56,20.32 v51.56,49.4
SPI_CIPO  (via drill 0.3, 0.38)
  Top 0.203: J11.DO/DAT0 14.17,44.65 v14.22,44.7 14.22,43.69 15.11,42.8 v28.57,42.8 43.56,42.8 44.2,43.43 44.2,45.03 U3.12 | J15.64 27.54,26.82 27.93,27.21 v27.93,27.32
  Bottom 0.203: J5.3 14.22,56.9 v14.22,44.7 | v27.93,27.32 28.57,27.97 v28.57,42.8
SPI_COPI  (via drill 0.3, 0.38)
  Top 0.203: U3.13 45.59,46.02 45.81,45.81 45.81,43.52 44.7,42.42 43.31,42.42 42.62,41.73 29.79,41.73 v29.67,41.6 | J11.DI/CMD 14.48,40.25 14.77,40.54 17.14,40.54 v17.4,40.28 18.69,38.99 v29.72,38.99 | v29.21,26.67 28.86,26.32 J15.62
  Bottom 0.203: v29.21,26.67 29.59,27.05 29.59,38.86 v29.72,38.99 29.84,39.12 29.84,41.43 v29.67,41.6 | J5.2 16.51,51.56 17.4,50.67 v17.4,40.28
SPI_SCK  (via drill 0.3, 0.38)
  Top 0.203: v28.32,25.65 27.71,25.65 27.55,25.82 J15.60 | v43.5,44.13 U3.11 | J11.SCLK 10.76,42.45 11.18,42.04 v19.05,42.04 26.14,42.04 28.42,39.75 v29.18,39.75 30.33,40.89 31.17,40.89 31.6,41.33 43.12,41.33 v43.5,41.71
  Bottom 0.203: J5.1 v19.05,42.04 | v28.32,25.65 28.32,26.8 28.96,27.43 28.96,39.52 v29.18,39.75 | v43.5,41.71 v43.5,44.13
SWDCK
  Top 0.203: J2.4 16.76,20.7 16.76,17.27 17.97,16.07 J15.21
SWDIO
  Top 0.203: J2.2 17.14,21.59 17.14,17.53 18.1,16.57 J15.23
  Bottom 0.203: J2.2 16.51,23.5 TP1.P$1
TX1  (via drill 0.3)
  Top 0.203: v23.24,13.03 21.2,15.07 J15.17 | v27.96,4.06 39.24,4.06 40.64,2.67 J6.1
  Bottom 0.203: v23.24,13.03 27.96,8.31 v27.96,4.06
TX2  (via drill 0.3)
  Top 0.203: v29.97,16.89 28.07,16.89 27.5,16.32 J15.22
  Bottom 0.203: v29.97,16.89 31.11,15.75 31.11,3.17 J12.1
USB_D+  (via drill 0.3)
  Top 0.203: J1.B6 5.32,9.41 5.21,9.53 5.21,10.16 | J1.A6 5.33,10.41 5.21,10.29 5.21,10.16 | 5.21,10.16 v4.74,10.16 | v15.75,11.3 17.4,11.3 17.67,11.57 J15.3
  Bottom 0.203: v4.74,10.16 5.37,10.79 15.24,10.79 v15.75,11.3
USB_D-  (via drill 0.3)
  Top 0.203: J1.A7 6.74,9.91 6.86,10.03 6.86,10.67 6.62,10.91 J1.B7 4.9,10.91 v4.74,11.08 | v15.33,12.05 15.35,12.07 J15.5
  Bottom 0.203: v4.74,11.08 4.95,11.29 14.57,11.29 v15.33,12.05
V_USB
  Top 0.254: J1.VBUS1 5.36,12.61 5.17,12.42 4.32,12.42 4.09,12.42 4.06,12.39 4.06,8.26 4.42,7.9 5.17,7.9 5.36,7.71 J1.VBUS2
  Top 0.61: BYP.1 3.28,20.19 2.79,20.19 2.31,19.71 F2.1 2.31,15.34 2.92,14.73 2.92,13.21 3.71,12.42 4.32,12.42
VIN  (via drill 0.3, 0.38)
  Top 0.203: R5.2 17.44,9.31 v17.65,9.53 | v20.83,12.45 20.2,13.07 J15.9 17.79,13.07 17.53,13.34 17.02,13.34 16.87,13.19 13.34,13.19 | 13.34,13.19 R10.2 | BYP.2 4.22,21.34 4.85,21.97 9.27,21.97 v9.4,22.1 | 13.34,13.19 9.33,13.19 9.31,13.21 | JP2.2 11.56,29.21 12.06,28.7 v12.06,28.07
  Top 0.559: U5.8 9.19,12.04 9.31,12.17
  Top 0.61: BYP.2 4.7,20.32 5.33,19.68 5.33,17.8 F2.2 C2.+ 7.49,16.39 8.38,15.49 C1.1 C13.1 9.31,13.21 9.31,12.17
  Bottom 0.203: v17.65,9.53 19.56,9.53 20.95,10.92 20.95,12.32 v20.83,12.45 | v12.06,28.07 9.4,25.4 v9.4,22.1
VIN/3
  Top 0.203: J15.49 17.57,23.07 16.64,24 13.97,24 13.34,23.37 R10.1 R9.2
VREG_EN  (via drill 0.3)
  Top 0.203: D1.C 13.24,11.01 R5.1 12.7,12.19 12.32,12.57 11.05,12.57 | 11.05,12.57 v10.54,12.57 | U5.5 11.13,12.49 11.05,12.57
  Bottom 0.203: v10.54,12.57 9.75,13.36 JP6.2
WDIR  (via drill 0.38)
  Top 0.203: J13.2 52.07,27.3 50.05,25.28 D10.C 47.29,25.28 R14.1 46.69,25.28 D9.A v43.2,25.28 v43.19,25.27 | J15.38 40.95,20.32 v41.1,20.17
  Bottom 0.203: v41.1,20.17 43.19,22.27 v43.19,25.27
WSPEED  (via drill 0.3)
  Top 0.203: J13.3 49.74,28.57 R16.1 | R16.1 C12.2 47.96,31.87 D8.C | R16.1 47.96,30.36 D5.A 36.7,30.35 v36.45,30.1 | J15.10 36.29,13.32 v36.4,13.21
  Bottom 0.203: v36.4,13.21 36.4,30.05 v36.45,30.1

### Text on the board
Bottom: v10
Dimension: ROUTE OUT | ROUTE OUT | ROUTE OUT
Measures: in | in | in | in
Document: Selective Solder Nozzle Width: / 0.354331
tDocu: Priyanka Makin

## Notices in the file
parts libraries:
SparkFun-Aesthetics: Licensing: Creative Commons ShareAlike 4.0 International - https://creativecommons.org/licenses/by-sa/4.0
SparkFun-Aesthetics: Released under the Creative Commons Attribution Share-Alike 4.0 License
SparkFun-Aesthetics: https://creativecommons.org/licenses/by-sa/4.0
